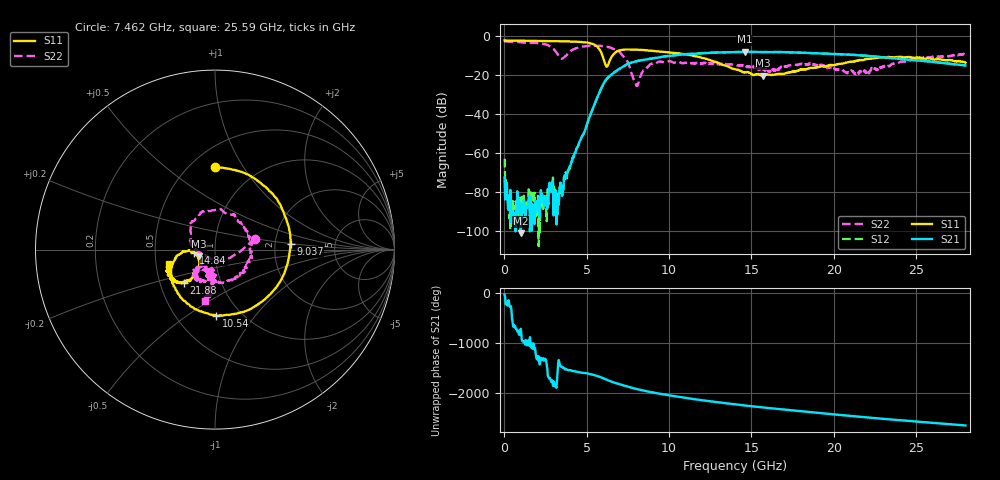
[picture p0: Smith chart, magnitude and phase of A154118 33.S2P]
!  2-Port S-parameters saved by WinCal
! VAR MeasName=S-Parameters (CALIBRATED_DATA) read from VNA (N5230A)
! VAR MeasDate=2015-9-10 14:36:56
! VAR NAME=A154118 33
! VAR FILENAME=A154118 33.S2P
! VAR DATE=2015-9-10 14:36:56
! VAR PHYS_PORTS=1,2
# Hz S DB R 50
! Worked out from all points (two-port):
!   801 points, 10 MHz to 28 GHz, reference 50 ohm
!   highest |S21| = -7.97 dB at 14.6 GHz (marker M1); lowest = -100.9 dB at 989.6 MHz (marker M2)
!   |S21| within 3 dB of the highest: 9.276 GHz to 23.26 GHz (13.98 GHz wide, 86 % of centre)
!   lowest |S11| = -20.2 dB at 15.68 GHz (marker M3), VSWR 1.22, Z = 41.6 - j3.06 ohm
!   |S11| at or under -10 dB: 5.96 GHz to 6.554 GHz (593.8 MHz wide, 9.49 % of centre); 11.46 GHz to end of sweep
!   |S22| runs from -25.5 to -2.7 dB; largest |S21 - S12| = 0.0079
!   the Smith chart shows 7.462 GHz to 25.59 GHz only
!   S11 on the Smith chart (normalised r, x): 7.462 GHz: 0.65, +0.76; 9.037 GHz: 2.44, +0.19; 10.54 GHz: 0.77, -0.66; 14.84 GHz: 0.79, -0.03; 21.88 GHz: 0.66, -0.26; 25.59 GHz: 0.59, -0.10
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1e7  -2.15 179.7  -72.41 -24.9  -62.71 -125.8  -2.67 179.8
3.248875e8  -2.19 175.2  -89.48 90.4  -81.32 10.7  -2.72 172.1
9.8965e8  -2.33 166.7  -100.89 6.5  -83.67 -175.1  -3.09 155.6
2.5291e9  -2.46 145.9  -85.67 94.5  -81.62 59.7  -4.18 100.5
3.193862e9  -2.51 134.9  -90.39 57.0  -80.91 20.1  -8.70 25.6
3.753662e9  -2.59 123.8  -72.48 -87.2  -71.44 -97.1  -9.81 -108.6
4.698325e9  -3.00 98.2  -51.60 -159.5  -51.48 -158.2  -5.29 166.7
6.132812e9  -14.51 -64.7  -22.79 72.0  -22.70 71.9  -5.35 103.2
7.462338e9  -6.77 90.3  -14.28 -74.8  -14.27 -75.0  -12.78 15.4
8.022138e9  -6.85 62.2  -12.78 -124.7  -12.81 -124.8  -25.49 -102.0
9.036775e9  -7.49 4.4  -11.29 163.8  -11.25 163.8  -13.80 128.8
9.351662e9  -7.76 -16.1  -10.92 144.5  -10.84 144.6  -13.08 111.3
1.054124e10  -8.68 -89.0  -9.59 78.6  -9.49 78.2  -13.11 61.5
1.4005e10  -16.94 -178.5  -8.13 -74.0  -8.11 -74.6  -14.66 -82.1
1.459979e10  -18.41 -177.2  -7.97 -96.6  -7.97 -96.9  -15.37 -90.2
1.48447e10  -18.50 -171.7  -8.02 -106.0  -7.98 -106.9  -15.70 -101.4
1.56844e10  -20.19 -158.1  -8.10 -135.8  -8.12 -136.4  -16.11 -104.5
1.869332e10  -16.12 -130.7  -8.60 124.2  -8.63 123.7  -13.97 -119.6
2.187719e10  -11.89 -133.4  -9.92 27.4  -9.87 26.9  -17.46 -102.6
2.334666e10  -10.70 -146.2  -11.04 -15.0  -10.99 -16.1  -15.29 -90.9
2.558586e10  -11.51 -162.7  -12.72 -75.7  -12.75 -76.4  -10.67 -101.2
2.8e10  -13.51 -163.4  -14.93 -138.9  -14.97 -139.8  -8.81 -112.9
